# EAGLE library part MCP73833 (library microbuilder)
Lithium-Polymer/Lithium-Ion Battery Charger [Part No.] Microchip MCP73833 MSOP10 (tube only): Digikey: MCP73833T-AMI/UN or MCP73833-FCI/UN-ND Mouser: 579-MCP73833-AMI/UN DFN10 (tape): Digikey: Note Chips ending in 'AMI' have no timer, and chips ending in 'FCI' have a 6-hour timer that will end the charge sequence after 6 horus regqrdless of current charge level.
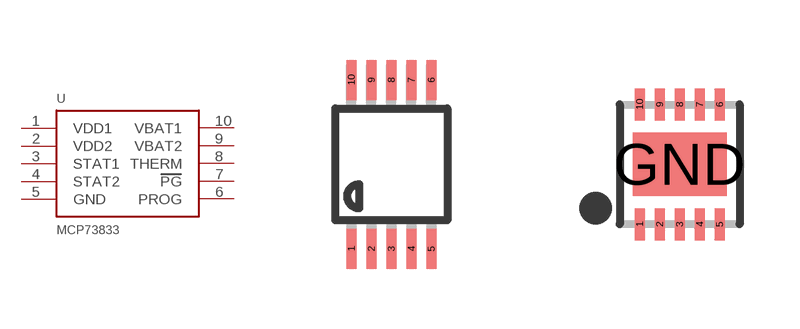
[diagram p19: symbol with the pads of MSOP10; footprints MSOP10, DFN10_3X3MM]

Designator prefix U

## MCP73833  [MSOP10]
1  VDD1
2  VDD2
3  STAT1
4  STAT2
5  GND
6  PROG
7  PG
8  THERM
9  VBAT2
10  VBAT1

## MCP73833DFN  [DFN10_3X3MM]
1  VDD1
2  VDD2
3  STAT1
4  STAT2
5  GND
6  PROG
7  PG
8  THERM
9  VBAT1
10  VBAT2

## Footprint MSOP10 (pad centres in mm)
10-Lead Mini Small Outline Package [MSOP]
smd 0.25 x 1: 1 -1,-2.113; 2 -0.5,-2.113; 3 0,-2.113; 4 0.5,-2.113; 5 1,-2.113; 6 1,2.113; 7 0.5,2.113; 8 0,2.113; 9 -0.5,2.113; 10 -1,2.113

## Footprint DFN10_3X3MM (pad centres in mm)
10-Lead 3.3mm DFN Source: http://ww1.microchip.com/downloads/en/DeviceDoc/22005b.pdf
smd 0.25 x 0.8: 1 -1,-1.5; 2 -0.5,-1.5; 3 0,-1.5; 4 0.5,-1.5; 5 1,-1.5; 6 1,1.5; 7 0.5,1.5; 8 0,1.5; 9 -0.5,1.5; 10 -1,1.5
smd 2.35 x 1.58: GND 0,0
